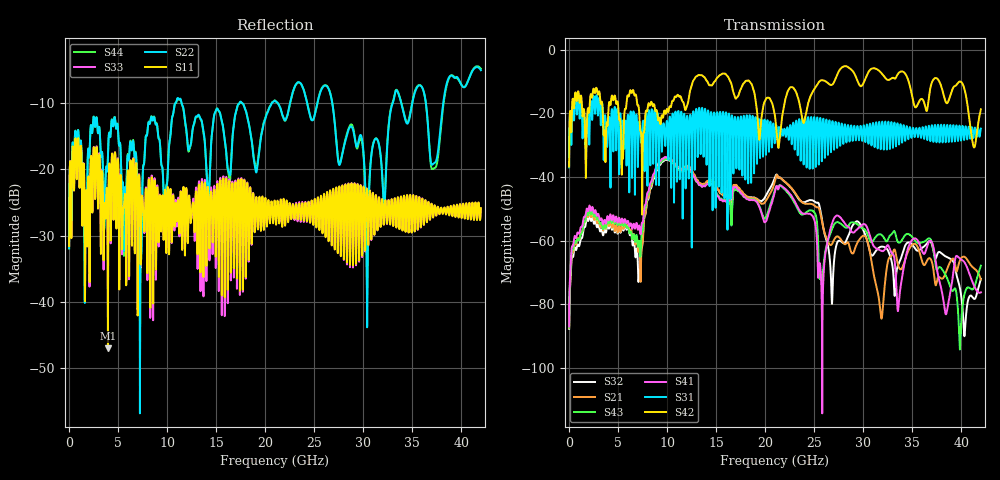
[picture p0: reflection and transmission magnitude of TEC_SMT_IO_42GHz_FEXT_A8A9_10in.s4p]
!! CHANNEL DESCRIPTION: Next Generation 28Gbps High Density SMT I/O Connector
!!  with 10" 5-6-5 Megatron 6 Stripline trace on host side and 1.25" 7-5-7 Megtron 6 Microstrip trace on plug side at 14GHz
!! HOST PCB DESCRIPTION: PCB thickness 2.86 mm, Nelco 4000-13SI (Dk 3.32, Df 0.010)
!!  23 Layer Board, 12 GND planes, 2 Layer route-out on Layers 10,12, 8 mil stub on vias
!!  Pairs on following layers
!!  Layer 10 - A8A9
!! CONNECTOR DESCRIPTION:  Next Generation 28Gbps High Density SMT I/O Connector
!! PLUG-IN CARD DESCRIPTION:  PCB thickness 1mm thick, Nelco 4000-13SI (Dk 3.32, Df 0.010)
!!  6 Layer Board, 4 GND planes, 0.35 x 1.4mm mating pads
!!  Micro-strip diff traces referenced to GND plane 3mils down, 2nd GND plane 15mils from top of board
!!  PCB GND planes are symmetric
!! MODEL DESCRIPTION: TE Connectivity S-parameter model produced from Macro-model
!! MODEL DATE: 9/25/2014 CR1a_GC1i, VR6&12_4
!! MODEL STATUS: Developmental
!! MODEL GEOMETRY: 2 Rows - Rows A, B. 3 pairs in each row, 6 total pairs
!! MODEL FREQUENCY RANGE: DC to 42 GHz in 10 MHz frequency steps
!! MODEL EDGE RATE LIMITATION: 11.90 ps (Using conservative 0.5/Fmax rule of thumb)
!! TIME-DOMAIN TRANSFORM CAUTIONS:
!! 1.) Do not simulate transient edge rates faster than the number listed above.  Edge
!!  rates faster than this number contain significant spectral content at frequencies
!!  above the model's highest frequency.
!! 2.) Even when simulating edge rates that are slower than the number listed above, be
!!  aware that the best time resolution possible with a direct iFFT is (1 / 2Fmax).
!!  As a result, time resolution is typically not adequate for most time-domain
!!  simulations unless tricks such as frequency-domain zero-padding and windowing are
!!  used to minimize leakage and aliasing.
!! 3.) Because the model has a uniform frequency step, a direct iFFT will result in an
!!  impulse that that has a time length given by either (1 / Fstep) or (1 / 2Fstep),
!!  depending on the transform being used.  Care has been taken in selecting the
!!  frequency step to ensure a settled impulse response for the model.  Therefore,
!!  convolution with the model's impulse response should present no issues.  However,
!!  if directly concatenating s-parameter models in the frequency domain a user must
!!  either interpolate necessary interim frequencies or complete impulse response
!!  zero-padding.  Impulse response zero-padding is more difficult, but more accurate.
!! PORT DEFINITIONS:
!! Port  1  ----->  Host, Bot Row  A8  B5  Module, Top Row  <-----  Port  2
!! Port  3  ----->  Host, Bot Row  A9  B6  Module, Top Row  <-----  Port  4
# Hz S MA R 50
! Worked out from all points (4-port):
!   4200 points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, 10 MHz to 42 GHz, reference 50 ohm
!   strongest paths, dB at 10 MHz, 10.51 GHz, 21.01 GHz, 31.51 GHz, 42 GHz:
!     S42: -36.7, -16.2, -21.0, -6.3, -18.7
!     S31: -36.9, -21.9, -28.5, -28.5, -24.8
!     S41: -87.0, -34.9, -44.4, -62.7, -76.3
!     S43: -87.3, -35.4, -43.9, -58.1, -67.9
!     S21: -87.5, -35.0, -41.1, -76.6, -72.2
!     S32: -87.7, -35.5, -40.1, -62.4, -72.0
!   lowest |S11| = -47.0 dB at 3.97 GHz (marker M1), VSWR 1.01, Z = 50.3 + j0.344 ohm
!   |S11| at or under -10 dB: start of sweep to end of sweep
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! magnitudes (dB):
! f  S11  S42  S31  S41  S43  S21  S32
! 10 MHz  -31.6  -36.7  -36.9  -87.0  -87.3  -87.5  -87.7
! 3.97 GHz  -47.0  -22.2  -26.1  -52.6  -53.9  -54.0  -55.1
! 7.19 GHz  -22.0  -21.5  -22.7  -55.7  -61.0  -62.0  -70.2
! 9.98 GHz  -26.2  -18.6  -22.3  -33.8  -34.3  -34.0  -34.6
! 25.7 GHz  -24.0  -9.6  -24.4  -71.6  -72.2  -52.4  -51.6
! 30.42 GHz  -24.5  -7.7  -24.1  -56.0  -57.8  -60.0  -60.2
! 42 GHz  -25.9  -18.7  -24.8  -76.3  -67.9  -72.2  -72.0
